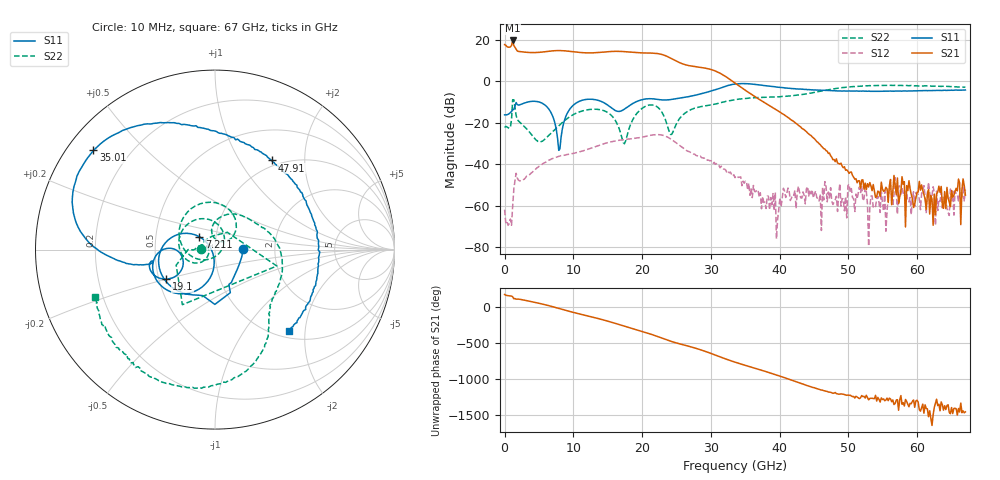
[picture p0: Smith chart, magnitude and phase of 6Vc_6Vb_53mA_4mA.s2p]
! MARKI MICROWAVE INC.
! Date:  05/05/2020
! Model Number:  APM-7099CH
! Description:  2-port Small Signal S-parameter data for APM-7099CH
! Frequency Range:  10 MHz to 67 GHz
! Port Configuration:  PORT 1: Input
!  PORT 2: Output
! Bias Condition: Vc = +6V, Vb = +6V
! APM-7099CH s2p files are only valid for small signal conditions (below -5 dBm input power)
!S2P File: Measurements: Mag<S11> Ang<S11>, Mag<S21> Ang<S21>, Mag<S12> Ang<S12>, Mag<S22> Ang<S22>!row 1
# Hz S  dB  R 50
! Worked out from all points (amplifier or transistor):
!   401 points, 10 MHz to 67 GHz, reference 50 ohm
!   highest |S21| = 19.6 dB at 1.182 GHz (marker M1)
!   |S21| within 3 dB of that: start of sweep to 355.7 MHz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
!   unconditionally stable (mu >= 1): start of sweep to end of sweep
!   at 11.06 GHz: K = 4.37, MAG = 14.5 dB, |S12| = -33.9 dB
!   at 33.51 GHz: K = 27.16, MAG = 5.4 dB, |S12| = -46.5 dB
!   at 67 GHz: K = 34616.21, MAG = -49.7 dB, |S12| = -52.3 dB
!   S11 on the Smith chart (normalised r, x): 10 MHz: 1.36, +0.01; 7.211 GHz: 0.83, +0.12; 19.1 GHz: 0.55, -0.20; 35.01 GHz: 0.08, +0.35; 47.91 GHz: 0.91, +1.39; 67 GHz: 1.14, -1.65
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1e7  -16.24 0.9  17.60 178.7  -61.90 137.4  -22.34 179.5
1.182325e9  -13.78 -63.5  19.62 147.6  -60.07 82.2  -8.96 -14.9
1.68475e9  -10.30 -90.1  15.57 114.3  -44.36 -80.3  -16.52 180.0
4.531825e9  -9.71 -161.6  13.79 67.2  -42.36 -166.9  -28.20 168.3
7.211425e9  -18.87 140.6  14.67 4.1  -36.96 129.0  -23.62 -135.2
9.221125e9  -14.83 -102.8  14.47 -49.9  -35.28 84.3  -17.73 -144.7
1.123082e10  -9.25 -137.8  13.76 -99.1  -33.72 48.1  -14.42 -174.8
1.508275e10  -11.73 178.4  14.22 166.5  -29.52 -32.3  -15.27 102.1
1.709245e10  -14.13 -154.7  14.31 109.0  -28.28 -81.6  -27.61 7.0
1.910215e10  -9.96 -148.8  13.80 51.5  -27.47 -129.9  -16.11 -173.6
2.094438e10  -8.44 -162.4  13.57 -2.1  -26.28 -177.7  -11.56 120.5
2.245165e10  -8.87 -169.7  13.17 -51.9  -25.77 133.4  -13.10 63.1
2.41264e10  -8.87 -167.9  11.13 -109.4  -27.74 75.4  -25.67 60.2
2.563368e10  -8.13 -167.8  8.66 -151.6  -31.38 35.3  -17.24 94.7
2.931812e10  -5.43 -173.2  6.18 103.8  -37.24 -29.1  -11.82 40.8
3.132782e10  -3.39 178.7  3.84 31.9  -41.71 -65.5  -10.42 22.4
3.3505e10  -1.36 157.8  -0.90 -41.6  -46.45 -98.7  -8.88 1.6
3.501228e10  -1.17 140.8  -4.38 -86.7  -48.17 -126.3  -8.32 -11.9
4.472582e10  -4.19 75.6  -26.83 -29.8  -52.37 -27.7  -5.62 -55.1
4.790785e10  -4.59 57.5  -37.76 -112.4  -58.25 -46.8  -3.70 -69.0
5.594665e10  -4.75 10.2  -50.47 178.3  -52.22 -108.2  -2.03 -112.5
6.7e10  -4.25 -47.4  -54.89 -13.3  -52.27 -97.1  -2.90 -158.5
